| IBIS file stm32h562_563_573_lqfp144.ibs
[IBIS ver] 4.2
[File name] stm32h562_563_573_lqfp144.ibs
[File Rev] 1.1
[Date] 07-05-2024
[Source] Data Created at STMicroelectronics
[Notes]  File originated from ELDO simulations.
[Disclaimer]  This information is for modeling purpose only and is
   not guaranteed. The information is subject to change without
   notice.
[Copyright] Copyright 2024 STMicroelectronics Inc.
|   stm32h562_563_573_lqfp144
[Component] stm32h562_563_573_lqfp144
[Manufacturer] STMicroelectronics
[Package]
| variable   typ   min   max
R_pkg  0  NA  NA
L_pkg  0  NA  NA
C_pkg  0  NA  NA
[Pin]   signal_name   model_name
1  PE2  io8_ft_i3c_spi
2  PE3  io8_ft_i3c_spi
3  PE4  io8_ft_i3c_spi
4  PE5  io8_ft_i3c_spi
5  PE6  io8_ft_i3c_spi
6  VBAT  power
7  PC13  io8_ft_i3c_spi
8  PC14-OSC32_IN  io8_ft_i3c_spi
9  PC15-OSC32_OUT  io8_ft_i3c_spi
10  PF0  io8_ft_i3c_spi
11  PF1  io8_ft_i3c_spi
12  PF2  io8_ft_i3c_spi
13  PF3  io8_ft_i3c_spi
14  PF4  io8_ft_i3c_spi
15  PF5  io8_ft_i3c_spi
16  VSS  gnd
17  VDD  power
18  PF6  io8_ft_i3c_spi
19  PF7  io8_ft_i3c_spi
20  PF8  io8_ft_i3c_spi
21  PF9  io8_ft_i3c_spi
22  PF10  io8_ft_i3c_spi
23  PH0-OSC_IN  io8_ft_i3c_spi
24  PH1-OSC_OUT  io8_ft_i3c_spi
25  NRST  ioreset_ft_v33
26  PC0  io8_ft_spi
27  PC1  io8_ft_spi
28  PC2  io8_ft_spi
29  PC3  io8_ft_spi
30  VDD  power
31  VSSA  nc
32  VREFP  nc
33  VDDA  nc
34  PA0  io8_ft_spi
35  PA1  io8_ft_spi_tamp
36  PA2  io8_ft_spi
37  PA3  io8_ft_spi
38  VSS  gnd
39  VDD  power
40  PA4  io8_ft_spi
41  PA5  io8_ft_spi
42  PA6  io8_ft_spi
43  PA7  io8_ft_spi
44  PC4  io8_ft_spi
45  PC5  io8_ft_spi
46  PB0  io8_ft_spi
47  PB1  io8_ft_spi
48  PB2  io8_ft_i3c_spi
49  PF11  io8_ft_spi
50  PF12  io8_ft_spi
51  VSS  gnd
52  VDD  power
53  PF13  io8_ft_spi
54  PF14  io8_ft_spi
55  PF15  io8_ft_i3c_spi
56  PG0  io8_ft_i3c_spi
57  PG1  io8_ft_i3c_spi
58  PE7  io8_ft_i3c_spi
59  PE8  io8_ft_i3c_spi
60  PE9  io8_ft_i3c_spi
61  VSS  gnd
62  VDD  power
63  PE10  io8_ft_i3c_spi
64  PE11  io8_ft_i3c_spi
65  PE12  io8_ft_i3c_spi
66  PE13  io8_ft_i3c_spi
67  PE14  io8_ft_i3c_spi
68  PE15  io8_ft_i3c_spi
69  PB10  io8_ft_i3c_spi
70  VCAP  nc
71  VSS  gnd
72  VDD  power
73  PB12  io8_ft_i3c_spi
74  PB13  nc
|io8usb_ft_pd
75  PB14  nc
|io8usb_ft_pd
76  PB15  io8_ft_spi
77  PD8  io8_ft_i3c_spi
78  PD9  io8_ft_i3c_spi
79  PD10  io8_ft_i3c_spi
80  PD11  io8_ft_i3c_spi
81  PD12  io8_ft_i3c_spi
82  PD13  io8_ft_i3c_spi
83  VSS  gnd
84  VDD  power
85  PD14  io8_ft_i3c_spi
86  PD15  io8_ft_i3c_spi
87  PG2  io8_ft_i3c_spi
88  PG3  io8_ft_i3c_spi
89  PG4  io8_ft_i3c_spi
90  PG5  io8_ft_i3c_spi
91  PG6  io8_ft_i3c_spi
92  PG7  io8_ft_i3c_spi
93  PG8  io8_ft_i3c_spi
94  VSS  gnd
95  VDD  power
96  PC6  io8_ft_i3c_spi
97  PC7  io8_ft_i3c_spi
98  PC8  io8_ft_i3c_spi
99  PC9  io8_ft_i3c_spi
100  PA8  io8_ft_i3c_spi
101  PA9  io8_ft_i3c_spi
102  PA10  io8_ft_i3c_spi
103  PA11  io8usb_ft_i3c_spi_phy
104  PA12  io8usb_ft_i3c_spi_phy
105  PA13  io8_ft_i3c_spi
106  VDDUSB  power
107  VSS  gnd
108  VDD  power
109  PA14  io8_ft_i3c_spi
110  PA15  io8_ft_i3c_spi
111  PC10  io8_ft_i3c_spi
112  PC11  io8_ft_i3c_spi
113  PC12  io8_ft_i3c_spi
114  PD0  io8_ft_i3c_spi
115  PD1  io8_ft_i3c_spi
116  PD2  io8_ft_i3c_spi
117  PD3  io8_ft_i3c_spi
118  PD4  io8_ft_i3c_spi
119  PD5  io8_ft_i3c_spi
120  VSS  gnd
121  VDDIO2  power
122  PD6  io8_ft_i3c_spi
123  PD7  io8_ft_i3c_spi
124  PG9  io8_ft_i3c_spi
125  PG10  io8_ft_i3c_spi
126  PG11  io8_ft_i3c_spi
127  PG12  io8_ft_i3c_spi
128  PG13  io8_ft_i3c_spi
129  PG14  io8_ft_i3c_spi
130  VSS  gnd
131  VDD  power
132  PG15  io8_ft_i3c_spi
133  PB3  io8_ft_i3c_spi
134  PB4  io8_ft_i3c_spi
135  PB5  io8_ft_i3c_spi
136  PB6  io8_ft_i3c_spi
137  PB7  io8_ft_i3c_spi
138  BOOT0  vpphv
139  PB8  io8_ft_i3c_spi
140  PB9  io8_ft_i3c_spi
141  PE0  io8_ft_i3c_spi
142  VCAP  nc
143  VSS  gnd
144  VDD  power
[Package Model]   484-lqfp-20x20-144-ldo-221014
[Pin Mapping]   pulldown_ref   pullup_ref   | Comment
1  gndio  vddiom
2  gndio  vddiom
3  gndio  vddiom
4  gndio  vddiom
5  gndio  vddiom
6  nc  vsw
7  gndio  vddiom  | Depending on IO usage
| 7  gndio  vsw  | Depending on IO usage
8  gndio  vddiom  | Depending on IO usage
| 8  gndio  vsw  | Depending on IO usage
9  gndio  vddiom  | Depending on IO usage
| 9  gndio  vsw  | Depending on IO usage
10  gndio  vddiom
11  gndio  vddiom
12  gndio  vddiom
13  gndio  vddiom
14  gndio  vddiom
15  gndio  vddiom
16  gndio  nc
17  nc  vddiom
18  gndio  vddiom
19  gndio  vddiom
20  gndio  vddiom
21  gndio  vddiom
22  gndio  vddiom
23  gndio  vddiom
24  gndio  vddiom
25  gndio  vddiom
26  gndio  vddiom
27  gndio  vddiom
28  gndio  vddiom
29  gndio  vddiom
30  nc  vddiom
31  nc  nc
32  nc  nc
33  nc  nc
34  gndio  vddiom
35  gndio  vddiom
36  gndio  vddiom
37  gndio  vddiom
38  gndio  nc
39  nc  vddiom
40  gndio  vddiom
41  gndio  vddiom
42  gndio  vddiom
43  gndio  vddiom
44  gndio  vddiom
45  gndio  vddiom
46  gndio  vddiom
47  gndio  vddiom
48  gndio  vddiom
49  gndio  vddiom
50  gndio  vddiom
51  gndio  nc
52  nc  vddiom
53  gndio  vddiom
54  gndio  vddiom
55  gndio  vddiom
56  gndio  vddiom
57  gndio  vddiom
58  gndio  vddiom
59  gndio  vddiom
60  gndio  vddiom
61  gndio  nc
62  nc  vddiom
63  gndio  vddiom
64  gndio  vddiom
65  gndio  vddiom
66  gndio  vddiom
67  gndio  vddiom
68  gndio  vddiom
69  gndio  vddiom
70  nc  nc
71  gndio  nc
72  nc  vddiom
73  gndio  vddiom
|74  gndio  vddiom
|75  gndio  vddiom
74 nc nc
75 nc nc
76  gndio  vddiom
77  gndio  vddiom
78  gndio  vddiom
79  gndio  vddiom
80  gndio  vddiom
81  gndio  vddiom
82  gndio  vddiom
83  gndio  nc
84  nc  vddiom
85  gndio  vddiom
86  gndio  vddiom
87  gndio  vddiom
88  gndio  vddiom
89  gndio  vddiom
90  gndio  vddiom
91  gndio  vddiom
92  gndio  vddiom
93  gndio  vddiom
94  gndio  nc
95  nc  vddiom
96  gndio  vddiom
97  gndio  vddiom
98  gndio  vddiom
99  gndio  vddiom
100  gndio  vddiom
101  gndio  vddiom  | Depending on IO usage
| 101  gndio  vddusb  | Depending on IO usage
102  gndio  vddiom  | Depending on IO usage
| 102  gndio  vddusb  | Depending on IO usage
103  gndio  vddiom  | Depending on IO usage
| 103  gndio  vddusb  | Depending on IO usage
104  gndio  vddiom  | Depending on IO usage
| 104  gndio  vddusb  | Depending on IO usage
105  gndio  vddiom  | Depending on IO usage
| 105  gndio  vddusb  | Depending on IO usage
106  nc  vddusb
107  gndio  nc
108  nc  vddiom
109  gndio  vddiom
110  gndio  vddiom
111  gndio  vddiom
112  gndio  vddiom
113  gndio  vddiom
114  gndio  vddiom
115  gndio  vddiom
116  gndio  vddiom
117  gndio  vddiom
118  gndio  vddiom
119  gndio  vddiom
120  gndio  nc
121  nc  vddmmc
122  gndio  vddiom  | Depending on IO usage
| 122  gndio  vddmmc  | Depending on IO usage
123  gndio  vddiom  | Depending on IO usage
| 123  gndio  vddmmc  | Depending on IO usage
124  gndio  vddiom  | Depending on IO usage
| 124  gndio  vddmmc  | Depending on IO usage
125  gndio  vddiom  | Depending on IO usage
| 125  gndio  vddmmc  | Depending on IO usage
126  gndio  vddiom  | Depending on IO usage
| 126  gndio  vddmmc  | Depending on IO usage
127  gndio  vddiom  | Depending on IO usage
| 127  gndio  vddmmc  | Depending on IO usage
128  gndio  vddiom  | Depending on IO usage
| 128  gndio  vddmmc  | Depending on IO usage
129  gndio  vddiom  | Depending on IO usage
| 129  gndio  vddmmc  | Depending on IO usage
130  gndio  nc
131  nc  vddiom
132  gndio  vddiom  | Depending on IO usage
| 132  gndio  vddmmc  | Depending on IO usage
133  gndio  vddiom  | Depending on IO usage
| 133  gndio  vddmmc  | Depending on IO usage
134  gndio  vddiom  | Depending on IO usage
| 134  gndio  vddmmc  | Depending on IO usage
135  gndio  vddiom  | Depending on IO usage
| 135  gndio  vddmmc  | Depending on IO usage
136  gndio  vddiom  | Depending on IO usage
| 136  gndio  vddmmc  | Depending on IO usage
137  gndio  vddiom  | Depending on IO usage
| 137  gndio  vddmmc  | Depending on IO usage
138  gndio  vddiom  | Depending on IO usage
| 138  gndio  vddmmc  | Depending on IO usage
139  gndio  vddiom  | Depending on IO usage
| 139  gndio  vddmmc  | Depending on IO usage
140  gndio  vddiom  | Depending on IO usage
| 140  gndio  vddmmc  | Depending on IO usage
141  gndio  vddiom  | Depending on IO usage
| 141  gndio  vddmmc  | Depending on IO usage
142  nc  nc
143  gndio  nc
144  nc  vddiom
[Model Selector] io8_ft_i3c_spi
io8_ft_spi_ls_1v2 "io8_ft spi low speed @ 1.2V"
io8_ft_spi_ls_1v8 "io8_ft spi low speed @ 1.8V"
io8_ft_spi_ls_3v3 "io8_ft spi low speed @ 3.3V"
io8_ft_spi_ms_1v2 "io8_ft spi med speed @ 1.2V"
io8_ft_spi_ms_1v8 "io8_ft spi med speed @ 1.8V"
io8_ft_spi_ms_3v3 "io8_ft spi med speed @ 3.3V"
io8_ft_spi_fs_1v2 "io8_ft spi fast speed @ 1.2V"
io8_ft_spi_fs_1v8 "io8_ft spi fast speed @ 1.8V"
io8_ft_spi_fs_3v3 "io8_ft spi fast speed @ 3.3V"
io8_ft_spi_hs_1v2 "io8_ft spi high speed @ 1.2V"
io8_ft_spi_hs_1v8 "io8_ft spi high speed @ 1.8V"
io8_ft_spi_hs_3v3 "io8_ft spi high speed @ 3.3V"
io8_ft_hslv_spi_ls_1v2 "io8_ft spi hslv low speed @ 1.2V"
io8_ft_hslv_spi_ls_1v8 "io8_ft spi hslv low speed @ 1.8V"
io8_ft_hslv_spi_ls_2v5 "io8_ft spi hslv low speed @ 2.5V"
io8_ft_hslv_spi_ms_1v2 "io8_ft spi hslv med speed @ 1.2V"
io8_ft_hslv_spi_ms_1v8 "io8_ft spi hslv med speed @ 1.8V"
io8_ft_hslv_spi_ms_2v5 "io8_ft spi hslv med speed @ 2.5V"
io8_ft_hslv_spi_fs_1v2 "io8_ft spi hslv fast speed @ 1.2V"
io8_ft_hslv_spi_fs_1v8 "io8_ft spi hslv fast speed @ 1.8V"
io8_ft_hslv_spi_fs_2v5 "io8_ft spi hslv fast speed @ 2.5V"
io8_ft_hslv_spi_hs_1v2 "io8_ft spi hslv high speed @ 1.2V"
io8_ft_hslv_spi_hs_1v8 "io8_ft spi hslv high speed @ 1.8V"
io8_ft_hslv_spi_hs_2v5 "io8_ft spi hslv high speed @ 2.5V"
io8_ft_i3c_spi_ls_1v2 "io8_ft i3c spi open-drain low speed @ 1.2V"
io8_ft_i3c_spi_ls_1v8 "io8_ft i3c spi open-drain low speed @ 1.8V"
io8_ft_i3c_spi_ls_3v3 "io8_ft i3c spi open-drain low speed @ 3.3V"
io8_ft_i3c_spi_ms_1v2 "io8_ft i3c spi open-drain med speed @ 1.2V"
io8_ft_i3c_spi_ms_1v8 "io8_ft i3c spi open-drain med speed @ 1.8V"
io8_ft_i3c_spi_ms_3v3 "io8_ft i3c spi open-drain med speed @ 3.3V"
io8_ft_i3c_spi_fs_1v2 "io8_ft i3c spi open-drain fast speed @ 1.2V"
io8_ft_i3c_spi_fs_1v8 "io8_ft i3c spi open-drain fast speed @ 1.8V"
io8_ft_i3c_spi_fs_3v3 "io8_ft i3c spi open-drain fast speed @ 3.3V"
io8_ft_i3c_spi_hs_1v2 "io8_ft i3c spi open-drain high speed @ 1.2V"
io8_ft_i3c_spi_hs_1v8 "io8_ft i3c spi open-drain high speed @ 1.8V"
io8_ft_i3c_spi_hs_3v3 "io8_ft i3c spi open-drain high speed @ 3.3V"
io8_ft_hslv_i3c_spi_ls_1v2 "io8_ft hslv i3c spi open-drain low speed @ 1.2V"
io8_ft_hslv_i3c_spi_ls_1v8 "io8_ft hslv i3c spi open-drain low speed @ 1.8V"
io8_ft_hslv_i3c_spi_ls_2v5 "io8_ft hslv i3c spi open-drain low speed @ 2.5V"
io8_ft_hslv_i3c_spi_ms_1v2 "io8_ft hslv i3c spi open-drain med speed @ 1.2V"
io8_ft_hslv_i3c_spi_ms_1v8 "io8_ft hslv i3c spi open-drain med speed @ 1.8V"
io8_ft_hslv_i3c_spi_ms_2v5 "io8_ft hslv i3c spi open-drain med speed @ 2.5V"
io8_ft_hslv_i3c_spi_fs_1v2 "io8_ft hslv i3c spi open-drain fast speed @ 1.2V"
io8_ft_hslv_i3c_spi_fs_1v8 "io8_ft hslv i3c spi open-drain fast speed @ 1.8V"
io8_ft_hslv_i3c_spi_fs_2v5 "io8_ft hslv i3c spi open-drain fast speed @ 2.5V"
io8_ft_hslv_i3c_spi_hs_1v2 "io8_ft hslv i3c spi open-drain high speed @ 1.2V"
io8_ft_hslv_i3c_spi_hs_1v8 "io8_ft hslv i3c spi open-drain high speed @ 1.8V"
io8_ft_hslv_i3c_spi_hs_2v5 "io8_ft hslv i3c spi open-drain high speed @ 2.5V"
io8_ft_i3c_fmp_spi_3v3 "io8_ft i3c fm+ spi open-drain @ 3.3V"
io8_ft_i3c_fmp_spi_1v8 "io8_ft i3c fm+ spi open-drain @ 1.8V"
io8_ft_i3c_fmp_spi_1v2 "io8_ft i3c fm+ spi open-drain @ 1.2V"
[Model Selector] io8_ft_spi
io8_ft_spi_ls_1v2 "io8_ft spi low speed @ 1.2V"
io8_ft_spi_ls_1v8 "io8_ft spi low speed @ 1.8V"
io8_ft_spi_ls_3v3 "io8_ft spi low speed @ 3.3V"
io8_ft_spi_ms_1v2 "io8_ft spi med speed @ 1.2V"
io8_ft_spi_ms_1v8 "io8_ft spi med speed @ 1.8V"
io8_ft_spi_ms_3v3 "io8_ft spi med speed @ 3.3V"
io8_ft_spi_fs_1v2 "io8_ft spi fast speed @ 1.2V"
io8_ft_spi_fs_1v8 "io8_ft spi fast speed @ 1.8V"
io8_ft_spi_fs_3v3 "io8_ft spi fast speed @ 3.3V"
io8_ft_spi_hs_1v2 "io8_ft spi high speed @ 1.2V"
io8_ft_spi_hs_1v8 "io8_ft spi high speed @ 1.8V"
io8_ft_spi_hs_3v3 "io8_ft spi high speed @ 3.3V"
io8_ft_hslv_spi_ls_1v2 "io8_ft spi hslv low speed @ 1.2V"
io8_ft_hslv_spi_ls_1v8 "io8_ft spi hslv low speed @ 1.8V"
io8_ft_hslv_spi_ls_2v5 "io8_ft spi hslv low speed @ 2.5V"
io8_ft_hslv_spi_ms_1v2 "io8_ft spi hslv med speed @ 1.2V"
io8_ft_hslv_spi_ms_1v8 "io8_ft spi hslv med speed @ 1.8V"
io8_ft_hslv_spi_ms_2v5 "io8_ft spi hslv med speed @ 2.5V"
io8_ft_hslv_spi_fs_1v2 "io8_ft spi hslv fast speed @ 1.2V"
io8_ft_hslv_spi_fs_1v8 "io8_ft spi hslv fast speed @ 1.8V"
io8_ft_hslv_spi_fs_2v5 "io8_ft spi hslv fast speed @ 2.5V"
io8_ft_hslv_spi_hs_1v2 "io8_ft spi hslv high speed @ 1.2V"
io8_ft_hslv_spi_hs_1v8 "io8_ft spi hslv high speed @ 1.8V"
io8_ft_hslv_spi_hs_2v5 "io8_ft spi hslv high speed @ 2.5V"
[Model Selector] io8_ft_spi_tamp
io8_ft_spi_ls_1v2 "io8_ft spi low speed @ 1.2V"
io8_ft_spi_ls_1v8 "io8_ft spi low speed @ 1.8V"
io8_ft_spi_ls_3v3 "io8_ft spi low speed @ 3.3V"
io8_ft_spi_ms_1v2 "io8_ft spi med speed @ 1.2V"
io8_ft_spi_ms_1v8 "io8_ft spi med speed @ 1.8V"
io8_ft_spi_ms_3v3 "io8_ft spi med speed @ 3.3V"
io8_ft_spi_fs_1v2 "io8_ft spi fast speed @ 1.2V"
io8_ft_spi_fs_1v8 "io8_ft spi fast speed @ 1.8V"
io8_ft_spi_fs_3v3 "io8_ft spi fast speed @ 3.3V"
io8_ft_spi_hs_1v2 "io8_ft spi high speed @ 1.2V"
io8_ft_spi_hs_1v8 "io8_ft spi high speed @ 1.8V"
io8_ft_spi_hs_3v3 "io8_ft spi high speed @ 3.3V"
io8_ft_hslv_spi_ls_1v2 "io8_ft spi hslv low speed @ 1.2V"
io8_ft_hslv_spi_ls_1v8 "io8_ft spi hslv low speed @ 1.8V"
io8_ft_hslv_spi_ls_2v5 "io8_ft spi hslv low speed @ 2.5V"
io8_ft_hslv_spi_ms_1v2 "io8_ft spi hslv med speed @ 1.2V"
io8_ft_hslv_spi_ms_1v8 "io8_ft spi hslv med speed @ 1.8V"
io8_ft_hslv_spi_ms_2v5 "io8_ft spi hslv med speed @ 2.5V"
io8_ft_hslv_spi_fs_1v2 "io8_ft spi hslv fast speed @ 1.2V"
io8_ft_hslv_spi_fs_1v8 "io8_ft spi hslv fast speed @ 1.8V"
io8_ft_hslv_spi_fs_2v5 "io8_ft spi hslv fast speed @ 2.5V"
io8_ft_hslv_spi_hs_1v2 "io8_ft spi hslv high speed @ 1.2V"
io8_ft_hslv_spi_hs_1v8 "io8_ft spi hslv high speed @ 1.8V"
io8_ft_hslv_spi_hs_2v5 "io8_ft spi hslv high speed @ 2.5V"
io8_ft_tamp_v33_1v2 "io8_ft tamp V33 @ 1.2V"
io8_ft_tamp_v33_1v8 "io8_ft tamp V33 @ 1.2V"
io8_ft_tamp_v33_3v3 "io8_ft tamp V33 @ 1.2V"
[Model Selector] io8usb_ft_i3c_spi_phy
io8_ft_spi_ls_1v2 "io8_ft spi low speed @ 1.2V"
io8_ft_spi_ls_1v8 "io8_ft spi low speed @ 1.8V"
io8_ft_spi_ls_3v3 "io8_ft spi low speed @ 3.3V"
io8_ft_spi_ms_1v2 "io8_ft spi med speed @ 1.2V"
io8_ft_spi_ms_1v8 "io8_ft spi med speed @ 1.8V"
io8_ft_spi_ms_3v3 "io8_ft spi med speed @ 3.3V"
io8_ft_spi_fs_1v2 "io8_ft spi fast speed @ 1.2V"
io8_ft_spi_fs_1v8 "io8_ft spi fast speed @ 1.8V"
io8_ft_spi_fs_3v3 "io8_ft spi fast speed @ 3.3V"
io8_ft_spi_hs_1v2 "io8_ft spi high speed @ 1.2V"
io8_ft_spi_hs_1v8 "io8_ft spi high speed @ 1.8V"
io8_ft_spi_hs_3v3 "io8_ft spi high speed @ 3.3V"
io8_ft_hslv_spi_ls_1v2 "io8_ft spi hslv low speed @ 1.2V"
io8_ft_hslv_spi_ls_1v8 "io8_ft spi hslv low speed @ 1.8V"
io8_ft_hslv_spi_ls_2v5 "io8_ft spi hslv low speed @ 2.5V"
io8_ft_hslv_spi_ms_1v2 "io8_ft spi hslv med speed @ 1.2V"
io8_ft_hslv_spi_ms_1v8 "io8_ft spi hslv med speed @ 1.8V"
io8_ft_hslv_spi_ms_2v5 "io8_ft spi hslv med speed @ 2.5V"
io8_ft_hslv_spi_fs_1v2 "io8_ft spi hslv fast speed @ 1.2V"
io8_ft_hslv_spi_fs_1v8 "io8_ft spi hslv fast speed @ 1.8V"
io8_ft_hslv_spi_fs_2v5 "io8_ft spi hslv fast speed @ 2.5V"
io8_ft_hslv_spi_hs_1v2 "io8_ft spi hslv high speed @ 1.2V"
io8_ft_hslv_spi_hs_1v8 "io8_ft spi hslv high speed @ 1.8V"
io8_ft_hslv_spi_hs_2v5 "io8_ft spi hslv high speed @ 2.5V"
io8_ft_i3c_spi_ls_1v2 "io8_ft i3c spi open-drain low speed @ 1.2V"
io8_ft_i3c_spi_ls_1v8 "io8_ft i3c spi open-drain low speed @ 1.8V"
io8_ft_i3c_spi_ls_3v3 "io8_ft i3c spi open-drain low speed @ 3.3V"
io8_ft_i3c_spi_ms_1v2 "io8_ft i3c spi open-drain med speed @ 1.2V"
io8_ft_i3c_spi_ms_1v8 "io8_ft i3c spi open-drain med speed @ 1.8V"
io8_ft_i3c_spi_ms_3v3 "io8_ft i3c spi open-drain med speed @ 3.3V"
io8_ft_i3c_spi_fs_1v2 "io8_ft i3c spi open-drain fast speed @ 1.2V"
io8_ft_i3c_spi_fs_1v8 "io8_ft i3c spi open-drain fast speed @ 1.8V"
io8_ft_i3c_spi_fs_3v3 "io8_ft i3c spi open-drain fast speed @ 3.3V"
io8_ft_i3c_spi_hs_1v2 "io8_ft i3c spi open-drain high speed @ 1.2V"
io8_ft_i3c_spi_hs_1v8 "io8_ft i3c spi open-drain high speed @ 1.8V"
io8_ft_i3c_spi_hs_3v3 "io8_ft i3c spi open-drain high speed @ 3.3V"
io8_ft_hslv_i3c_spi_ls_1v2 "io8_ft hslv i3c spi open-drain low speed @ 1.2V"
io8_ft_hslv_i3c_spi_ls_1v8 "io8_ft hslv i3c spi open-drain low speed @ 1.8V"
io8_ft_hslv_i3c_spi_ls_2v5 "io8_ft hslv i3c spi open-drain low speed @ 2.5V"
io8_ft_hslv_i3c_spi_ms_1v2 "io8_ft hslv i3c spi open-drain med speed @ 1.2V"
io8_ft_hslv_i3c_spi_ms_1v8 "io8_ft hslv i3c spi open-drain med speed @ 1.8V"
io8_ft_hslv_i3c_spi_ms_2v5 "io8_ft hslv i3c spi open-drain med speed @ 2.5V"
io8_ft_hslv_i3c_spi_fs_1v2 "io8_ft hslv i3c spi open-drain fast speed @ 1.2V"
io8_ft_hslv_i3c_spi_fs_1v8 "io8_ft hslv i3c spi open-drain fast speed @ 1.8V"
io8_ft_hslv_i3c_spi_fs_2v5 "io8_ft hslv i3c spi open-drain fast speed @ 2.5V"
io8_ft_hslv_i3c_spi_hs_1v2 "io8_ft hslv i3c spi open-drain high speed @ 1.2V"
io8_ft_hslv_i3c_spi_hs_1v8 "io8_ft hslv i3c spi open-drain high speed @ 1.8V"
io8_ft_hslv_i3c_spi_hs_2v5 "io8_ft hslv i3c spi open-drain high speed @ 2.5V"
io8_ft_i3c_fmp_spi_3v3 "io8_ft i3c fm+ spi open-drain @ 3.3V"
io8_ft_i3c_fmp_spi_1v8 "io8_ft i3c fm+ spi open-drain @ 1.8V"
io8_ft_i3c_fmp_spi_1v2 "io8_ft i3c fm+ spi open-drain @ 1.2V"
io8usb_ft_phy_ls_2v5 "iousb ft low speed @ 2.5V"
io8usb_ft_phy_ls_3v3 "iousb ft low speed @ 3.3V"
io8usb_ft_phy_fs_2v5 "iousb ft fast speed @ 2.5V"
io8usb_ft_phy_fs_3v3 "iousb ft fast speed @ 3.3V"
[Model Selector] ioreset_ft_v33
ioreset_ft_v33_1v2 "Reset PAD. 5V tolerant. 1.2V range"
ioreset_ft_v33_1v8 "Reset PAD. 5V tolerant. 1.8V range"
ioreset_ft_v33_3v3 "Reset PAD. 5V tolerant. 3.3V range"
[Model Selector] vpphv
vpphv_1v2 "Flash Test cell v33 = 1.2 V range"
vpphv_1v8 "Flash Test cell v33 = 1.8 V range"
vpphv_3v3 "Flash Test cell v33 = 3.3 V range"
[Define Package Model]  484-lqfp-20x20-144-ldo-221014
[Manufacturer]  Unknown
[OEM]  Unknown
[Description]  None
[Number Of Pins]  137
[Pin Numbers]
| Pin Num   Terminal Name
138 | BOOT0
25 | NRST
34 | PA0
35 | PA1
36 | PA2
37 | PA3
40 | PA4
41 | PA5
42 | PA6
43 | PA7
100 | PA8
101 | PA9
102 | PA10
103 | PA11
104 | PA12
105 | PA13
109 | PA14
110 | PA15
46 | PB0
47 | PB1
48 | PB2
133 | PB3
134 | PB4
135 | PB5
136 | PB6
137 | PB7
139 | PB8
140 | PB9
69 | PB10
73 | PB12
74 | PB13
75 | PB14
76 | PB15
26 | PC0
27 | PC1
28 | PC2
29 | PC3
44 | PC4
45 | PC5
96 | PC6
97 | PC7
98 | PC8
99 | PC9
111 | PC10
112 | PC11
113 | PC12
7 | PC13
8 | PC14-OSC32_IN
9 | PC15-OSC32_OUT
114 | PD0
115 | PD1
116 | PD2
117 | PD3
118 | PD4
119 | PD5
122 | PD6
123 | PD7
77 | PD8
78 | PD9
79 | PD10
80 | PD11
81 | PD12
82 | PD13
85 | PD14
86 | PD15
141 | PE0
1 | PE2
2 | PE3
3 | PE4
4 | PE5
5 | PE6
58 | PE7
59 | PE8
60 | PE9
63 | PE10
64 | PE11
65 | PE12
66 | PE13
67 | PE14
68 | PE15
10 | PF0
11 | PF1
12 | PF2
13 | PF3
14 | PF4
15 | PF5
18 | PF6
19 | PF7
20 | PF8
21 | PF9
22 | PF10
49 | PF11
50 | PF12
53 | PF13
54 | PF14
55 | PF15
56 | PG0
57 | PG1
87 | PG2
88 | PG3
89 | PG4
90 | PG5
91 | PG6
92 | PG7
93 | PG8
124 | PG9
125 | PG10
126 | PG11
127 | PG12
128 | PG13
129 | PG14
132 | PG15
23 | PH0-OSC_IN
24 | PH1-OSC_OUT
6 | VBAT
70 | VCAP
142 | VCAP
72 | VDD
108 | VDD
17 | VDD
30 | VDD
39 | VDD
52 | VDD
62 | VDD
144 | VDD
84 | VDD
131 | VDD
95 | VDD
121 | VDDIO2
106 | VDDUSB
33 | VDDA
32 | VREFP
51 | VSS
130 | VSS
94 | VSS
16 | VSS
31 | VSSA
|[Merged Pins]  16
|38  |  VSS
|61  |  VSS
|71  |  VSS
|83  |  VSS
|107  |  VSS
|120  |  VSS
|143  |  VSS
[Model Data]
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[End Model Data]
[End Package Model]
|End [Component]
| Models and submodels in the file (64): io8_ft_hslv_i3c_spi_fs_1v2 (I/O_open_drain), io8_ft_hslv_i3c_spi_fs_1v8 (I/O_open_drain), io8_ft_hslv_i3c_spi_fs_2v5 (I/O_open_drain), io8_ft_hslv_i3c_spi_hs_1v2 (I/O_open_drain), io8_ft_hslv_i3c_spi_hs_1v8 (I/O_open_drain), io8_ft_hslv_i3c_spi_hs_2v5 (I/O_open_drain), io8_ft_hslv_i3c_spi_ls_1v2 (I/O_open_drain), io8_ft_hslv_i3c_spi_ls_1v8 (I/O_open_drain), io8_ft_hslv_i3c_spi_ls_2v5 (I/O_open_drain), io8_ft_hslv_i3c_spi_ms_1v2 (I/O_open_drain), io8_ft_hslv_i3c_spi_ms_1v8 (I/O_open_drain), io8_ft_hslv_i3c_spi_ms_2v5 (I/O_open_drain), io8_ft_hslv_spi_fs_1v2 (I/O), io8_ft_hslv_spi_fs_1v8 (I/O), io8_ft_hslv_spi_fs_2v5 (I/O), io8_ft_hslv_spi_hs_1v2 (I/O), io8_ft_hslv_spi_hs_1v8 (I/O), io8_ft_hslv_spi_hs_2v5 (I/O), io8_ft_hslv_spi_ls_1v2 (I/O), io8_ft_hslv_spi_ls_1v8 (I/O), io8_ft_hslv_spi_ls_2v5 (I/O), io8_ft_hslv_spi_ms_1v2 (I/O), io8_ft_hslv_spi_ms_1v8 (I/O), io8_ft_hslv_spi_ms_2v5 (I/O), io8_ft_i3c_fmp_spi_1v2 (I/O_open_drain), io8_ft_i3c_fmp_spi_1v8 (I/O_open_drain), io8_ft_i3c_fmp_spi_3v3 (I/O_open_drain), io8_ft_i3c_spi_fs_1v2 (I/O_open_drain), io8_ft_i3c_spi_fs_1v8 (I/O_open_drain), io8_ft_i3c_spi_fs_3v3 (I/O_open_drain), io8_ft_i3c_spi_hs_1v2 (I/O_open_drain), io8_ft_i3c_spi_hs_1v8 (I/O_open_drain), io8_ft_i3c_spi_hs_3v3 (I/O_open_drain), io8_ft_i3c_spi_ls_1v2 (I/O_open_drain), io8_ft_i3c_spi_ls_1v8 (I/O_open_drain), io8_ft_i3c_spi_ls_3v3 (I/O_open_drain), io8_ft_i3c_spi_ms_1v2 (I/O_open_drain), io8_ft_i3c_spi_ms_1v8 (I/O_open_drain), io8_ft_i3c_spi_ms_3v3 (I/O_open_drain), io8_ft_spi_fs_1v2 (I/O), io8_ft_spi_fs_1v8 (I/O), io8_ft_spi_fs_3v3 (I/O), io8_ft_spi_hs_1v2 (I/O), io8_ft_spi_hs_1v8 (I/O), io8_ft_spi_hs_3v3 (I/O), io8_ft_spi_ls_1v2 (I/O), io8_ft_spi_ls_1v8 (I/O), io8_ft_spi_ls_3v3 (I/O), io8_ft_spi_ms_1v2 (I/O), io8_ft_spi_ms_1v8 (I/O), io8_ft_spi_ms_3v3 (I/O), io8_ft_tamp_v33_1v2 (I/O), io8_ft_tamp_v33_1v8 (I/O), io8_ft_tamp_v33_3v3 (I/O), io8usb_ft_phy_fs_2v5 (I/O), io8usb_ft_phy_fs_3v3 (I/O), io8usb_ft_phy_ls_2v5 (I/O), io8usb_ft_phy_ls_3v3 (I/O), ioreset_ft_v33_1v2 (I/O_open_drain), ioreset_ft_v33_1v8 (I/O_open_drain), ioreset_ft_v33_3v3 (I/O_open_drain), vpphv_1v2 (Input), vpphv_1v8 (Input), vpphv_3v3 (Input)
